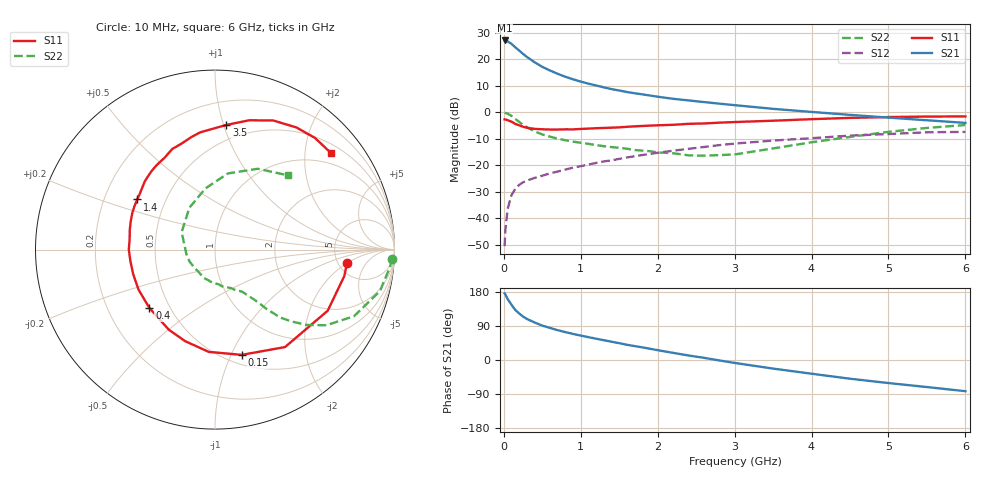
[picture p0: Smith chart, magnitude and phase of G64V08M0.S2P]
! SIEMENS Small Signal Semiconductors
! BFG193
! Si NPN RF Bipolar Junction Transistor in SOT223
! VCE = 4 V  IC = 8 mA
! Common Emitter S-Parameters:  August  1996
# GHz  S  MA  R  50
!  f  S11  S21  S12  S22
! GHz  MAG  ANG  MAG  ANG  MAG  ANG  MAG  ANG
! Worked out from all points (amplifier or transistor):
!   36 points, 10 MHz to 6 GHz, reference 50 ohm
!   highest |S21| = 27.1 dB at 10 MHz (marker M1)
!   |S21| within 3 dB of that: start of sweep to 165.6 MHz
!   unconditionally stable (mu >= 1): 956.8 MHz to 2.514 GHz
!   at 250 MHz: K = 0.47, MSG = 24.2 dB, |S12| = -26.4 dB
!   at 1.4 GHz: K = 1.08, MAG = 11.7 dB, |S12| = -18.1 dB
!   at 6 GHz: K = 0.87, MSG = 1.7 dB, |S12| = -7.3 dB
!   S11 on the Smith chart (normalised r, x): 10 MHz: 5.99, -2.01; 150 MHz: 0.59, -1.10; 400 MHz: 0.39, -0.33; 1.4 GHz: 0.34, +0.26; 3.5 GHz: 0.38, +1.02; 6 GHz: 0.71, +2.59
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0.01  0.7395 -5.9  22.78 175.8  0.003 93.0  0.9876 -2.9
0.02  0.7353 -11.6  22.62 172.8  0.006 81.7  0.9792 -5.8
0.05  0.7143 -28.5  21.83 160.5  0.0152 75.3  0.9479 -14.1
0.1  0.6687 -54.3  19.63 145.7  0.0277 66.9  0.8587 -25.6
0.15  0.605 -75.8  16.84 131.8  0.0364 57.6  0.7499 -34.2
0.2  0.5709 -93.5  14.65 122.7  0.043 53.6  0.6617 -39.4
0.25  0.5364 -108.1  12.7 114.5  0.0481 49.7  0.5809 -43.4
0.3  0.515 -120.0  11.13 108.3  0.0518 48.6  0.5256 -46.1
0.4  0.4893 -138.3  8.841 99.0  0.0582 46.9  0.4393 -49.0
0.5  0.4809 -152.4  7.241 90.8  0.064 46.6  0.384 -50.6
0.6  0.4759 -163.1  6.174 84.6  0.0709 46.7  0.3486 -52.2
0.7  0.4757 -172.0  5.357 78.7  0.0768 46.9  0.3212 -53.9
0.9  0.4791 173.0  4.215 68.8  0.0908 47.1  0.2809 -56.9
1.1  0.4951 161.5  3.486 60.3  0.104 46.9  0.2553 -62.7
1.4  0.5156 147.2  2.752 48.3  0.1249 44.5  0.2219 -71.8
1.7  0.5458 135.7  2.3 36.7  0.1491 41.8  0.1956 -83.2
2.2  0.5841 118.7  1.808 18.9  0.1895 33.9  0.1699 -111.0
2.8  0.6408 101.8  1.465 -1.1  0.2415 22.9  0.1567 -155.1
3.5  0.6974 84.8  1.168 -22.7  0.2944 7.3  0.2095 152.5
4.5  0.7892 65.7  0.899 -49.4  0.3652 -12.7  0.345 98.9
5.5  0.8349 48.2  0.711 -71.4  0.422 -37.4  0.5097 62.1
6  0.841 39.8  0.635 -82.3  0.4292 -51.7  0.5787 45.7
